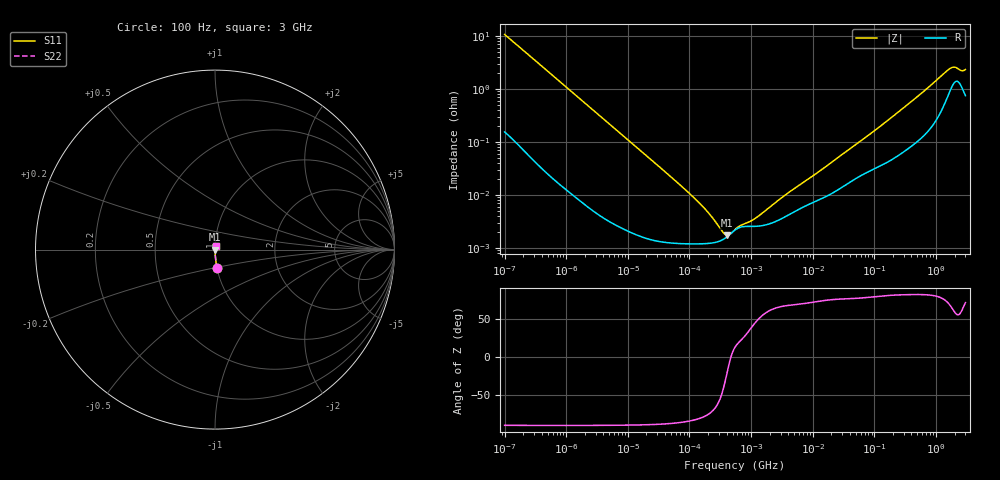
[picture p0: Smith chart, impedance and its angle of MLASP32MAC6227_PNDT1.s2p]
! MLASP32MAC6227_PNDT1  S-PARAMETER MODEL  ( Standard Model )
! Model Generated by TAIYO YUDEN Corporation (http://www.ty-top.com)
! Version 1.0
! TAIYO YUDEN Control No. 220601
! Copyright(c) 2014 TAIYO YUDEN CO.,LTD. All Rights Reserved.
! Product Description (link to TY-COMPAS)
! https://ds.yuden.co.jp/TYCOMPAS/or/detail?pn=MLASP32MAC6227MPNDT1&u=M
! Products Name : Multilayer Ceramic Capacitors
! Characteristics :
!  Capacitance : 220 [uF] , Rated Voltage : 2.5 [V] , TCC : X6S
!  Case Size : 3.2 x 2.5 / 0.126 x 0.098 [mm/inch] , Thickness : 2.5 / 0.098 [mm/inch]
!  (Conditions: Temperature = 25 [degC] , DC Bias Voltage = 0 [V])
! External Node Assignments :
!  1  o---| |---o  2
! GND o---------o GND
! Frequency Range : 100Hz  -  3GHz  [ 401 STEP ]
# MHZ S RI R 50
! Freq[MHz].  S11 Real  S11 Imag  S21 Real  S21 Imag  S12 Real  S12 Imag  S22 Real  S22 Imag
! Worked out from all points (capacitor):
!   401 points, 100 Hz to 3 GHz, reference 50 ohm
!   read as one part in series: C = 149 uF near 109 Hz
!   lowest |Z| = 1.74 mohm at 405.2 kHz (marker M1)
!   series resonance near 470.2 kHz, so ESL is about 770 pH
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0.0001  0.0128 -0.1052  0.9872 0.1052  0.9872 0.1052  0.0128 -0.1052
0.000114  0.0101 -0.0929  0.9899 0.0929  0.9899 0.0929  0.0101 -0.0929
0.000306  0.00167 -0.0352  0.9983 0.0352  0.9983 0.0352  0.00167 -0.0352
0.001788  0.00011 -0.0061  0.9999 0.0061  0.9999 0.0061  0.00011 -0.0061
0.031977  1.34e-05 -0.000345  1 0.000345  1 0.000345  1.34e-05 -0.000345
0.097915  1.2e-05 -0.000109  1 0.000109  1 0.000109  1.2e-05 -0.000109
0.106717  1.2e-05 -9.89e-05  1 9.89e-05  1 9.89e-05  1.2e-05 -9.89e-05
0.116311  1.2e-05 -8.98e-05  1 8.98e-05  1 8.98e-05  1.2e-05 -8.98e-05
0.405239  1.62e-05 -6.3e-06  1 6.3e-06  1 6.3e-06  1.62e-05 -6.3e-06
0.547723  2.18e-05 5.04e-06  1 -5.04e-06  1 -5.04e-06  2.18e-05 5.04e-06
3.486191  3.83e-05 8.99e-05  1 -8.99e-05  1 -8.99e-05  3.83e-05 8.99e-05
3.966702  4.16e-05 0.000101  1 -0.000101  1 -0.000101  4.16e-05 0.000101
9.794414  7.1e-05 0.000213  0.9999 -0.000213  0.9999 -0.000213  7.1e-05 0.000213
77.30952  0.000271 0.00127  0.9997 -0.00127  0.9997 -0.00127  0.000271 0.00127
175.1444  0.000443 0.00266  0.9996 -0.00266  0.9996 -0.00266  0.000443 0.00266
559.889  0.00121 0.00792  0.9988 -0.00792  0.9988 -0.00792  0.00121 0.00792
1642.185  0.0089 0.0218  0.9911 -0.0218  0.9911 -0.0218  0.0089 0.0218
1789.813  0.0111 0.0224  0.9889 -0.0224  0.9889 -0.0224  0.0111 0.0224
1950.712  0.0131 0.0219  0.9869 -0.0219  0.9869 -0.0219  0.0131 0.0219
2126.076  0.0142 0.0205  0.9858 -0.0205  0.9858 -0.0205  0.0142 0.0205
2525.516  0.0119 0.0186  0.9881 -0.0186  0.9881 -0.0186  0.0119 0.0186
3000  0.0079 0.0217  0.9921 -0.0217  0.9921 -0.0217  0.0079 0.0217
